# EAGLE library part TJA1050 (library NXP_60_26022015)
High speed CAN transceiver The TJA1050 is the interface between the Controller Area Network (CAN) protocol controller and the physical bus. The device provides differential transmit capability to the bus and differential receive capability to the CAN controller. The TJA1050 is the third Philips high-speed CAN transceiver after the PCA82C250 and the PCA82C251. The most important differences are: Much lower electromagnetic emission due to optimal matching of the output signals CANH and CANL Improved behaviour in case of an unpowered node No standby mode. This makes the TJA1050 eminently suitable for use in nodes that are in a power-down situation in partially powered networks. AAL Eindhoven MK
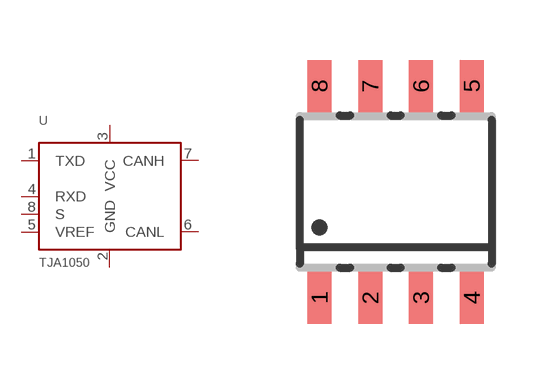
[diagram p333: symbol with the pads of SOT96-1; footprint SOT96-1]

Designator prefix U

## TJA1050  [SOT96-1]
1  TXD  out
2  GND
3  VCC
4  RXD
5  VREF  pas
6  CANL
7  CANH
8  S  pwr

## Footprint SOT96-1 (pad centres in mm)
SOT96-1 SO8: plastic small outline package; 8 leads; body width 3.9 mm JEDEC: MS-012 IEC: 076E03
smd 0.6 x 1.3: 1 -1.905,-2.65; 2 -0.635,-2.65; 3 0.635,-2.65; 4 1.905,-2.65; 5 1.905,2.65; 6 0.635,2.65; 7 -0.635,2.65; 8 -1.905,2.65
